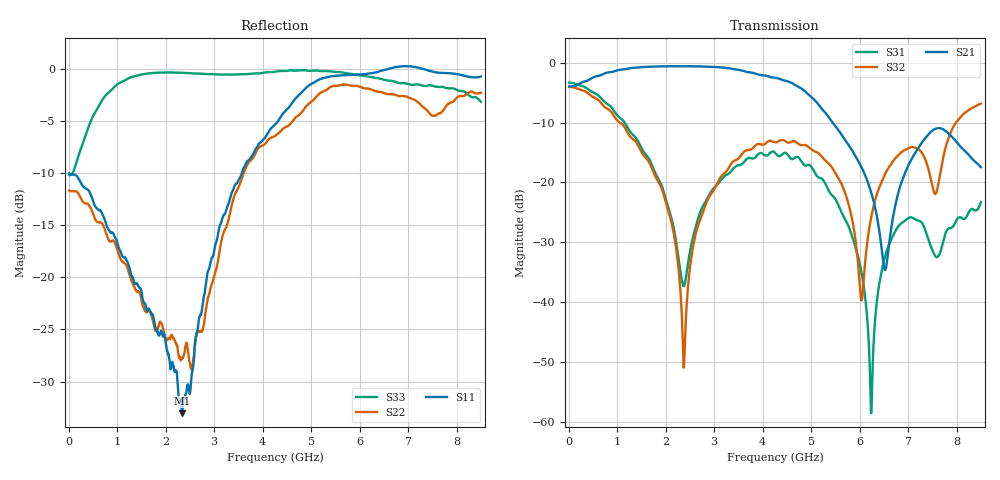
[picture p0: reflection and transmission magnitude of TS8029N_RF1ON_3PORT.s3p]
!Created with skrf (http://scikit-rf.org).
# GHz S RI R 50.0
!freq ReS11 ImS11 ReS12 ImS12 ReS13 ImS13
! ReS21 ImS21 ReS22 ImS22 ReS23 ImS23
! ReS31 ImS31 ReS32 ImS32 ReS33 ImS33
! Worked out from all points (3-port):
!   1601 points, 10 MHz to 8.5 GHz, reference 50 ohm
!   strongest paths, dB at 10 MHz, 2.132 GHz, 4.255 GHz, 6.378 GHz, 8.5 GHz:
!     S21: -4.0, -0.6, -2.5, -26.6, -17.5
!     S32: -4.1, -27.1, -13.3, -21.5, -6.9
!     S31: -3.3, -26.4, -15.1, -38.4, -23.3
!   lowest |S11| = -33.0 dB at 2.339 GHz (marker M1), VSWR 1.05, Z = 51.7 + j1.44 ohm
!   |S11| at or under -10 dB: start of sweep to 3.572 GHz
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0.01  -0.3143 0.00786  0.632 0.0011  0.6807 -0.0127
      0.6318 0.00105  -0.2608 0.00551  0.6265 -0.0106
      0.6805 -0.0128  0.6267 -0.0106  -0.3092 0.0202
0.6520563  -0.0822 0.1924  0.7758 -0.1112  0.2452 -0.4515
           0.7758 -0.1117  -0.0931 0.1576  0.2431 -0.4022
           0.2447 -0.4517  0.2432 -0.4022  0.4408 0.5177
1.883106  0.0526 0.0101  0.5486 -0.7518  -0.0678 -0.0751
          0.5486 -0.7516  0.0595 -0.0145  -0.0595 -0.0751
          -0.0677 -0.075  -0.0594 -0.0751  0.7803 -0.5544
2.339444  0.0174 0.0139  0.2984 -0.8851  -0.00215 -0.0146
          0.2983 -0.885  0.0242 -0.0326  -0.00677 -0.000545
          -0.0022 -0.0146  -0.00673 -0.000496  0.4957 -0.8163
4.255  0.474 0.2588  -0.6907 -0.2859  -0.0445 -0.1712
       -0.6896 -0.2865  -0.4598 -0.1227  0.1224 -0.1775
       -0.0446 -0.1709  0.1229 -0.1777  -0.737 -0.6254
5.767281  0.8299 -0.424  -0.1356 0.1558  -0.0426 0.00767
          -0.1358 0.1558  -0.1915 0.8115  -0.0454 -0.0489
          -0.0426 0.00766  -0.0455 -0.049  -0.8591 0.398
6.239537  0.784 -0.537  -0.0425 0.0703  -0.000643 -0.000975
          -0.0424 0.0702  0.2194 0.7626  0.051 -0.00591
          -0.000648 -0.000984  0.051 -0.00595  -0.5335 0.7385
6.653425  0.659 -0.7595  -0.0229 -0.0353  0.0102 -0.032
          -0.0228 -0.0352  0.6172 0.4334  0.126 -0.0686
          0.0102 -0.0319  0.126 -0.0685  -0.0763 0.8704
7.486506  0.4673 -0.8492  -0.2609 -0.058  -0.0193 -0.0203
          -0.262 -0.058  0.0416 -0.5952  0.0115 -0.0979
          -0.0193 -0.0203  0.0115 -0.0975  0.7957 0.2379
8.5  0.4803 -0.7811  -0.0714 0.1136  -0.0393 -0.0559
     -0.0715 0.1132  -0.2193 0.7339  0.0495 -0.4505
     -0.0393 -0.056  0.0486 -0.4513  0.0783 -0.6889
